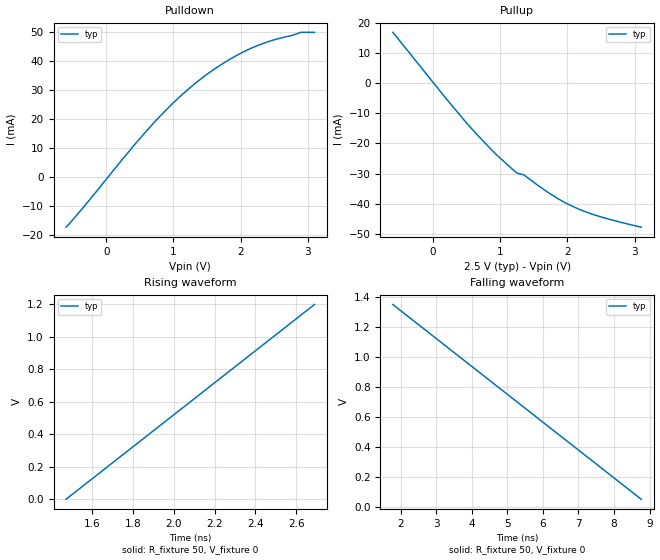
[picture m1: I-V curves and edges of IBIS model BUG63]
|********************* IBIS GOLDEN PARSER BUG REPORT FORM *********************
|INSTRUCTIONS
|To report a bug in the IBIS golden parser.  Please fill out the top part
|of the following form and send the complete form to ibischk-bug@vhdl.org.
|A list of reported bugs will be maintained on vhdl.org.
|PARSER VERSION NUMBER: 3.2.7
|PLATFORM (SPARC, HP700, PC, etc.): Sparc
|OS AND VERSION: Solaris 4.5
|REPORTED BY: Bob Ross
|DATE: 11/01/01
|DESCRIPTION OF BUG:
|Certain waveform test case percentage calculations are wrong.
|BUG47 introduced some more detailed reporting of waveform mismatch.
|Included were percentage differences since BUG47 changed the report
|to an error from warning if the mismatch was greater than 10%.  While
|the test seems to work in most cases, there are some cases where the
|reported percentage is wrong.
|The file below produces the following messages.  The Voltage difference
|calculation appears correct for the low side, and the internal percentages
|distinguishing between an Error and a Warning (10%) appear correct, but
|the REPORTED percentages of 100% and 176.4% are incorrect.  In the
|second case the percent difference should have been 2.3% making this
|"Warning" report correct inspite of reported percentage.  If this is changed
|to less than 2% error with the commented line at the end, the Warning
|message is correctly eliminated.  The reported percentages need to be fixed.
|Checking bug63.ibs for IBIS 3.2 Compatibility...
|ERROR - Model BUG63: The [Rising Waveform]
|   with [R_fixture]=50 Ohms and [V_fixture]=0V
|   has TYP column DC endpoints of  0.00V and  1.20v, but
|   an equivalent load applied to the model's I-V tables yields
|   different voltages ( 0.02V and  1.37V),
|   a difference of 100.00% and 12.65%, respectively.
|WARNING - Model BUG63: The [Falling Waveform]
|   with [R_fixture]=50 Ohms and [V_fixture]=0V
|   has TYP column DC endpoints of  0.05V and  1.35v, but
|   an equivalent load applied to the model's I-V tables yields
|   different voltages ( 0.02V and  1.37V),
|   a difference of 176.40% and  1.73%, respectively.
|Errors  : 1
|Warnings: 1
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[IBIS ver] 3.2
[File Name] bug63.ibs
[File Rev] 0.0
[Date] 10/31.01
[Source] Created
[Component] BUG63TEST
[Manufacturer] Anyone
[Package]
R_pkg 0 NA NA
L_pkg 0 NA NA
C_pkg 0 NA NA
[Pin] signal_name   model_name
D9   A35   BUG63
| Models and submodels in the file (1): BUG63 (I/O)
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[Model] BUG63
Model_type I/O
Vinh = 1.23V
Vinl = 1.21V
Rref = 500
Vref = 0
C_comp 4p 3p 6p
[Voltage Range] 2.5V NA NA
[Ramp]
|variable typ   min   max
 dV/dt_r  0.75/0.24n   NA   NA
 dV/dt_f  0.75/0.09n   NA   NA
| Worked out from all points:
|   slope of the pulldown table from 0 to 0.375 V, typ, clamps not added: 35.2 ohm
|   slope of the pullup table from 0 to 0.375 V, typ, clamps not added: 37 ohm
|   rising waveform, R_fixture 50, V_fixture 0: 20-80 % time 732ps typ, NA min, NA max; typ from 0 V to 1.2 V
|   falling waveform, R_fixture 50, V_fixture 0: 20-80 % time 4.19ns typ, NA min, NA max; typ from 1.35 V to 0.05 V
[Pulldown]
|Voltage   I(typ)   I(min)   I(max)
-600mV    -17.34mA   NA         NA
-350mV    -10.78mA   NA         NA
450mV     11.87mA    NA         NA
700mV     18.42mA    NA         NA
1V        25.54mA    NA         NA
1.35V     32.66mA    NA         NA
1.55V     36.15mA    NA         NA
1.8V      39.94mA    NA         NA
2V        42.53mA    NA         NA
2.25V     45.21mA    NA         NA
2.9V      49.78mA    NA         NA
3.1V      49.78mA    NA         NA
[Pullup]
|Voltage   I(typ)   I(min)   I(max)
-600mV    16.82mA    NA         NA
200mV     -5.32mA    NA         NA
550mV     -14.53mA   NA         NA
950mV     -23.89mA   NA         NA
1.25V     -29.87mA   NA         NA
1.35V     -30.42mA   NA         NA
1.75V     -36.82mA   NA         NA
1.95V     -39.46mA   NA         NA
2.15V     -41.59mA   NA         NA
2.5V      -44.38mA   NA         NA
3.1V      -47.76mA   NA         NA
[Rising Waveform]
R_fixture = 50
V_fixture = 0
|Time   V(typ)   V(min)   V(max)
1.47ns    0V         NA         NA
2.69ns    1.2V       NA         NA
[Falling Waveform]
R_fixture = 50
V_fixture = 0
|Time   V(typ)   V(min)   V(max)
1.78ns    1.35V      NA         NA
8.77ns    50mV       NA         NA
